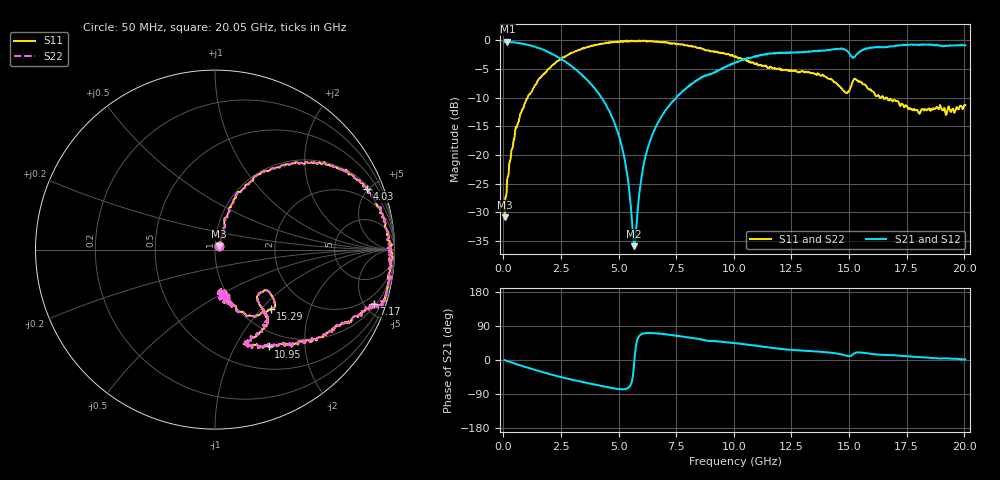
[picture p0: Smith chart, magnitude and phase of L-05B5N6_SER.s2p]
! P/N: L-05C5N6_SER
! Measured by Marlon
! Sep. 23, 2003
! Measure with a Series-through-fixture
#	mhz	s	ma	r	50
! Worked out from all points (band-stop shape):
!   1001 points, 50 MHz to 20.05 GHz, reference 50 ohm
!   highest |S21| = -0.25 dB at 170 MHz (marker M1); lowest = -35.9 dB at 5.67 GHz (marker M2)
!   |S21| within 3 dB of the highest: start of sweep to 2.487 GHz; 10.59 GHz to end of sweep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
!   lowest |S11| = -30.8 dB at 50 MHz (marker M3), VSWR 1.06, Z = 52.3 + j1.81 ohm
!   |S11| at or under -10 dB: start of sweep to 1.051 GHz; 16.49 GHz to 16.6 GHz (115.7 MHz wide, 0.699 % of centre); 16.64 GHz to end of sweep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
!   |S22| runs from -30.8 to -0.1 dB; largest |S21 - S12| = 0
!   S11 on the Smith chart (normalised r, x): 50 MHz: 1.05, +0.04; 4.03 GHz: 1.25, +4.88; 7.17 GHz: 1.21, -5.79; 10.95 GHz: 0.79, -1.38; 15.29 GHz: 1.35, -1.14; 20.05 GHz: 0.97, -0.56
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50  0.02868 37.2  0.9633 -0.3  0.9633 -0.3  0.02868 37.2
170  0.06284 56.3  0.9719 -3.1  0.9719 -3.1  0.06284 56.3
530  0.1724 72.0  0.9526 -10.6  0.9526 -10.6  0.1724 72.0
1030  0.3113 68.0  0.9127 -19.8  0.9127 -19.8  0.3113 68.0
2150  0.6076 50.4  0.7524 -39.6  0.7524 -39.6  0.6076 50.4
3390  0.8388 31.7  0.503 -57.6  0.503 -57.6  0.8388 31.7
4030  0.9095 21.8  0.3654 -65.8  0.3654 -65.8  0.9095 21.8
5110  0.9864 1.7  0.1255 -76.7  0.1255 -76.7  0.9864 1.7
5370  0.973 -3.3  0.06769 -75.2  0.06769 -75.2  0.973 -3.3
5670  0.9758 -6.1  0.01609 -12.0  0.01609 -12.0  0.9758 -6.1
6110  0.9926 -16.8  0.08692 70.2  0.08692 70.2  0.9926 -16.8
6730  0.9668 -19.3  0.1961 69.4  0.1961 69.4  0.9668 -19.3
7170  0.9348 -18.8  0.2641 67.1  0.2641 67.1  0.9348 -18.8
10050  0.7138 -45.7  0.6357 44.4  0.6357 44.4  0.7138 -45.7
10950  0.6168 -61.0  0.7169 37.1  0.7169 37.1  0.6168 -61.0
12150  0.5494 -72.2  0.7748 28.8  0.7748 28.8  0.5494 -72.2
13390  0.5165 -58.9  0.7994 23.2  0.7994 23.2  0.5165 -58.9
14890  0.3468 -45.7  0.8119 11.1  0.8119 11.1  0.3468 -45.7
15290  0.455 -46.9  0.7363 19.6  0.7363 19.6  0.455 -46.9
16730  0.2991 -75.9  0.8779 13.0  0.8779 13.0  0.2991 -75.9
18010  0.2364 -80.8  0.9146 7.9  0.9146 7.9  0.2364 -80.8
20050  0.271 -76.9  0.9033 1.4  0.9033 1.4  0.271 -76.9
